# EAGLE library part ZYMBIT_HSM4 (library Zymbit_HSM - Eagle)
Connector
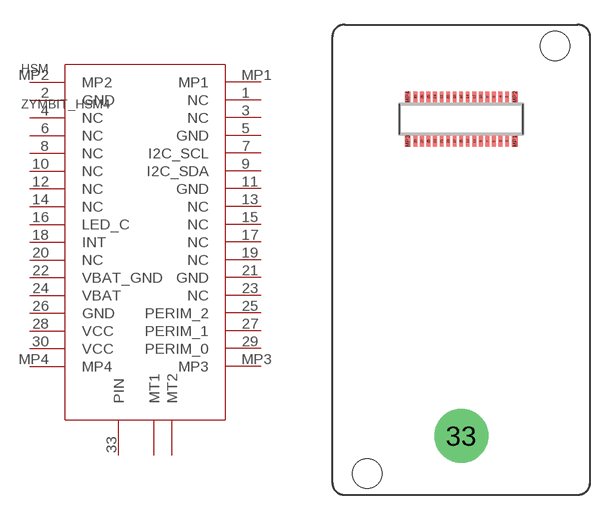
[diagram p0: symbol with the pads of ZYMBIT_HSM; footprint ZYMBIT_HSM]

Designator prefix HSM

## ZYMBIT_HSM4ZYMBIT_HSM4_ZYMBIT_HSM (DATASHEET_LINK: https://datasheet.lcsc.com/szlcsc/1909181103_Hirose-HRS-DF40C-30DP-0-4V-51_C429942.pdf; HEIGHT: 1.29mm; MANUFACTURER_NAME: HRS(Hirose); MANUFACTURER_PART_NUMBER: DF40C-30DP-0.4V(51))  [ZYMBIT_HSM]
1  NC  pas
2  GND  pas
3  NC  pas
4  NC  pas
5  GND  pas
6  NC  pas
7  I2C_SCL  pas
8  NC  pas
9  I2C_SDA  pas
10  NC  pas
11  GND  pas
12  NC  pas
13  NC  pas
14  NC  pas
15  NC  pas
16  LED_C  pas
17  NC  pas
18  INT  pas
19  NC  pas
20  NC  pas
21  GND  pas
22  VBAT_GND  pas
23  NC  pas
24  VBAT  pas
25  PERIM_2  pas
26  GND  pas
27  PERIM_1  pas
28  VCC  pas
29  PERIM_0  pas
30  VCC  pas
33  PIN  pas
MP1  MP1  pas
MP2  MP2  pas
MP3  MP3  pas
MP4  MP4  pas

## Footprint ZYMBIT_HSM (pad centres in mm)
smd 0.23 x 0.66: 1 2.8,-1.355; 2 2.8,1.355; 3 2.4,-1.355; 4 2.4,1.355; 5 2,-1.355; 6 2,1.355; 7 1.6,-1.355; 8 1.6,1.355; 9 1.2,-1.355; 10 1.2,1.355; 11 0.8,-1.355; 12 0.8,1.355; 13 0.4,-1.355; 14 0.4,1.355; 15 0,-1.355; 16 0,1.355; 17 -0.4,-1.355; 18 -0.4,1.355; 19 -0.8,-1.355; 20 -0.8,1.355; 21 -1.2,-1.355; 22 -1.2,1.355; 23 -1.6,-1.355; 24 -1.6,1.355; 25 -2,-1.355; 26 -2,1.355; 27 -2.4,-1.355; 28 -2.4,1.355; 29 -2.8,-1.355; 30 -2.8,1.355
drill 1.7 pad 3.3 round: 33 0,-19.371
smd 0.35 x 0.66: MP1 3.275,-1.355; MP2 3.275,1.355; MP3 -3.275,-1.355; MP4 -3.275,1.355
hole 1.8 at -5.73,-21.681
hole 1.8 at 5.73,4.459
